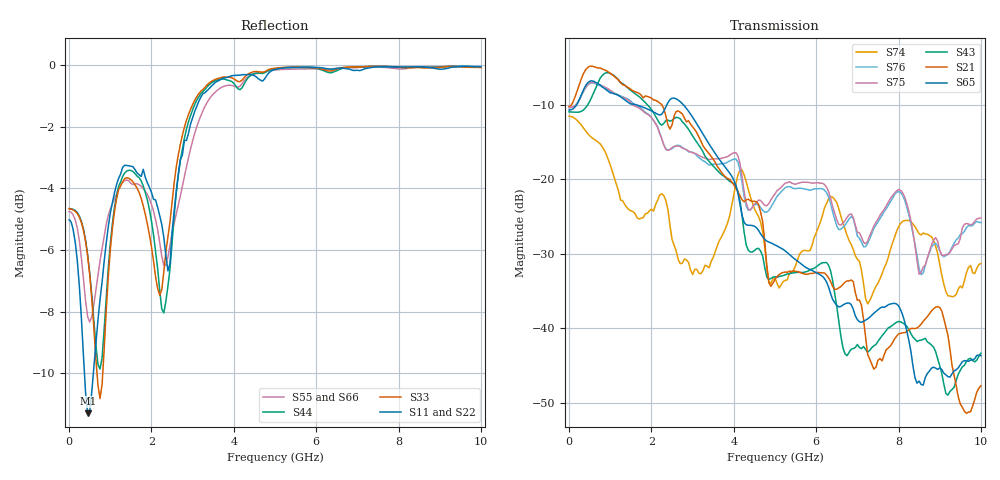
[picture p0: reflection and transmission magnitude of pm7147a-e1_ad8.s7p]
# GHz S DB R 50
! S-Parameters data
! Freq  dbS11  angS11  dbS12  angS12  dbS13  angS13  dbS14  angS14
!  dbS15  angS15  dbS16  angS16  dbS17  angS17  dbS21  angS21
!  dbS22  angS22  dbS23  angS23  dbS24  angS24  dbS25  angS25
!  dbS26  angS26  dbS27  angS27  dbS31  angS31  dbS32  angS32
!  dbS33  angS33  dbS34  angS34  dbS35  angS35  dbS36  angS36
!  dbS37  angS37  dbS41  angS41  dbS42  angS42  dbS43  angS43
!  dbS44  angS44  dbS45  angS45  dbS46  angS46  dbS47  angS47
!  dbS51  angS51  dbS52  angS52  dbS53  angS53  dbS54  angS54
!  dbS55  angS55  dbS56  angS56  dbS57  angS57  dbS61  angS61
!  dbS62  angS62  dbS63  angS63  dbS64  angS64  dbS65  angS65
!  dbS66  angS66  dbS67  angS67  dbS71  angS71  dbS72  angS72
!  dbS73  angS73  dbS74  angS74  dbS75  angS75  dbS76  angS76
!  dbS77  angS77
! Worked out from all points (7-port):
!   279 points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, 1 Hz to 10 GHz, reference 50 ohm
!   strongest paths, dB at 1 Hz, 7.943 MHz, 3.05 GHz, 6.55 GHz, 10 GHz:
!     S65: -10.7, -10.7, -12.1, -37.2, -43.7
!     S21: -10.2, -10.2, -13.3, -34.6, -47.7
!     S43: -11.0, -11.0, -14.6, -39.1, -43.4
!     S75: -10.4, -10.4, -16.5, -26.1, -25.2
!     S76: -10.4, -10.4, -16.6, -26.8, -25.8
!     S74: -11.6, -11.6, -32.1, -24.0, -31.3
!   lowest |S11| = -11.3 dB at 450 MHz (marker M1), VSWR 1.75, Z = 28.6 - j0.271 ohm
!   |S11| at or under -10 dB: 372.5 MHz to 588.7 MHz (216.3 MHz wide, 45 % of centre)
